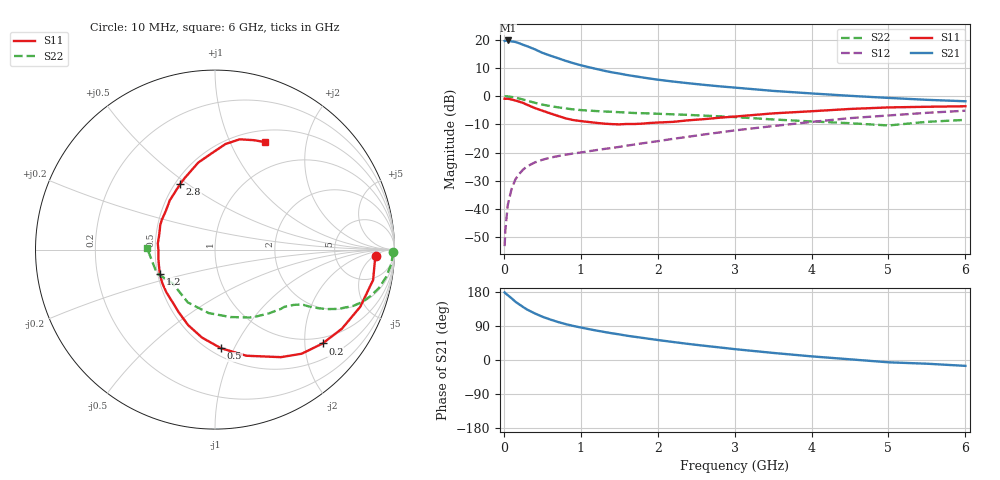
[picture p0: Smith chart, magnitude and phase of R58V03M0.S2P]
! SIEMENS Small Signal Semiconductors
! BFR183
! Si NPN RF Bipolar Junction Transistor in SOT23
! VCE = 8 V  IC = 3 mA
! Common Emitter S-Parameters:  May  1996
# GHz  S  MA  R  50
!  f  S11  S21  S12  S22
! GHz  MAG  ANG  MAG  ANG  MAG  ANG  MAG  ANG
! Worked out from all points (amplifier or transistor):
!   36 points, 10 MHz to 6 GHz, reference 50 ohm
!   highest |S21| = 19.7 dB at 50 MHz (marker M1)
!   |S21| within 3 dB of that: start of sweep to 391.1 MHz
!   unconditionally stable (mu >= 1): 1.289 GHz to 2.803 GHz
!   at 250 MHz: K = 0.29, MSG = 22.1 dB, |S12| = -26.1 dB
!   at 1.4 GHz: K = 1.04, MAG = 12.3 dB, |S12| = -18.4 dB
!   at 6 GHz: K = 0.88, MSG = 1.7 dB, |S12| = -5.2 dB
!   lowest NFmin = 1.10 dB at 450 MHz
!   S11 on the Smith chart (normalised r, x): 10 MHz: 17, -6; 200 MHz: 0.85, -2.41; 500 MHz: 0.56, -0.89; 1.2 GHz: 0.51, -0.16; 2.8 GHz: 0.53, +0.47; 6 GHz: 0.64, +1.36
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0.01  0.8998 -2.3  9.459 178.3  0.0022 89.0  0.9934 -0.9
0.02  0.8929 -4.4  9.561 176.2  0.0043 82.9  0.9905 -1.8
0.05  0.897 -10.9  9.649 171.2  0.0116 85.2  0.9853 -4.7
0.15  0.8332 -31.9  9.076 153.9  0.0334 73.2  0.9383 -13.2
0.2  0.7957 -41.1  8.611 146.8  0.0419 68.3  0.9037 -16.7
0.25  0.755 -50.2  8.079 139.9  0.0498 64.2  0.8691 -19.7
0.3  0.7028 -58.5  7.658 133.4  0.0567 61.1  0.8325 -22.1
0.4  0.6168 -73.5  6.755 123.2  0.0665 56.1  0.762 -25.7
0.5  0.5507 -86.5  5.835 114.3  0.0744 52.8  0.706 -28.0
0.6  0.4956 -98.4  5.216 107.1  0.0811 50.7  0.6664 -29.4
0.7  0.4465 -109.6  4.701 100.5  0.0862 49.9  0.6328 -30.5
0.8  0.404 -119.9  4.219 94.9  0.0915 49.3  0.6046 -31.4
0.9  0.3764 -129.0  3.835 90.0  0.096 49.5  0.5811 -32.0
1.1  0.3478 -147.8  3.254 81.7  0.1053 50.3  0.5535 -33.7
1.2  0.3357 -156.3  3.025 77.8  0.1103 50.6  0.5428 -34.5
1.6  0.3205 173.7  2.361 64.1  0.1324 53.1  0.5091 -38.4
2.2  0.3494 141.3  1.806 47.5  0.1749 55.2  0.4751 -46.7
2.8  0.413 118.2  1.489 33.3  0.2266 53.6  0.4382 -58.2
3.5  0.4937 100.9  1.235 18.7  0.2945 48.2  0.3853 -77.2
4.5  0.5912 84.3  1.01 1.8  0.4068 37.4  0.3308 -117.3
5.5  0.6463 70.7  0.858 -9.8  0.5051 24.3  0.3499 -158.0
6  0.66 65.3  0.809 -15.5  0.5504 15.8  0.3788 178.7
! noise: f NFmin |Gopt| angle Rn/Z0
0.45  1.1  0.37  35  0.3
0.9  1.15  0.34  85  0.23
1.8  1.9  0.35  160  0.13
